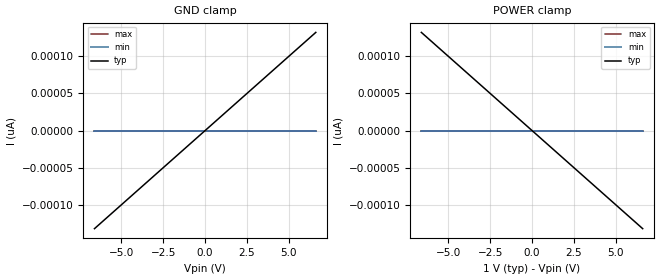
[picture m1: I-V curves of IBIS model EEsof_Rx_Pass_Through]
[IBIS Ver]   5.1
[File Name]   EEsof_Rx_Pass_Through.ibs
[File Rev]   1.0
[Component]   EEsof_Rx_Pass_Through
[Manufacturer] Keysight Technologies, Inc.
[Package]
R_pkg  0.0   NA   NA
L_pkg  0.0   NA   NA
C_pkg  0.0   NA   NA
[Pin]   signal_name   model_name   R_pin L_pin  C_pin
2p   EEsof_Rx_Pass_Through_2p   EEsof_Rx_Pass_Through
2n   EEsof_Rx_Pass_Through_2n   EEsof_Rx_Pass_Through
[Diff_Pin] inv_pin vdiff tdelay_typ tdelay_min tdelay_max
2p   2n   NA   NA   NA   NA
| Models and submodels in the file (1): EEsof_Rx_Pass_Through (Input)
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[Model] EEsof_Rx_Pass_Through
Model_type Input
C_comp 0p 0p 0p
Vinh = 0.25
Vinl = -0.25
[Temperature_Range] 25 125 0
[Voltage Range] 1.0 1.0 1.0
[Algorithmic Model]
Executable Windows_cl17.00.60315.1_64 EEsof_Rx_Pass_Through_x64.dll EEsof_Rx_Pass_Through.ami
Executable Linux_gcc4.6.2_64 EEsof_Rx_Pass_Through_x64.so EEsof_Rx_Pass_Through.ami
[End Algorithmic Model]
[GND Clamp]
-6.6V     -132pA     0A         0A
0V        0A         0A         0A
6.6V      132pA      0A         0A
[Power Clamp]
-6.6V     132pA      0A         0A
0V        0A         0A         0A
6.6V      -132pA     0A         0A
